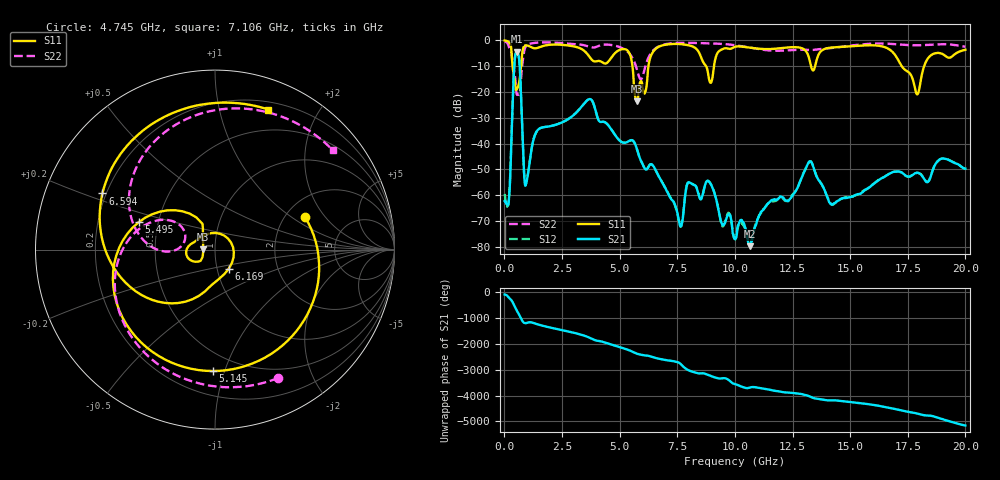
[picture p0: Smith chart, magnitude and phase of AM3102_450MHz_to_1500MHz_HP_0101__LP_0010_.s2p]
!Agilent Technologies,E8364B,MY43040894,A.07.50.67
!Agilent E8364B: A.07.50.67
!Date: Thursday, January 11, 2018 05:39:55
!Correction: S11(Full 2 Port(1,2))
!S21(Full 2 Port(1,2))
!S12(Full 2 Port(1,2))
!S22(Full 2 Port(1,2))
!S2P File: Measurements: S11, S21, S12, S22:
# Hz S  dB  R 50
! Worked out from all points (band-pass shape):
!   1601 points, 10 MHz to 20 GHz, reference 50 ohm
!   highest |S21| = -4.44 dB at 534.7 MHz (marker M1); lowest = -79.7 dB at 10.64 GHz (marker M2)
!   |S21| within 3 dB of the highest: 452.5 MHz to 642.6 MHz (190.1 MHz wide, 34.7 % of centre)
!   lowest |S11| = -23.6 dB at 5.745 GHz (marker M3), VSWR 1.14, Z = 43.8 + j0.156 ohm
!   |S11| at or under -10 dB: 355.8 MHz to 725.3 MHz (369.5 MHz wide, 68.3 % of centre); 5.555 GHz to 6.249 GHz (693.9 MHz wide, 11.8 % of centre); 17.24 GHz to 18.21 GHz (973.4 MHz wide, 5.49 % of centre)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
!   |S22| runs from -21.1 to -0.4 dB; largest |S21 - S12| = 0.0012
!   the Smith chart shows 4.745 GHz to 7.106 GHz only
!   S11 on the Smith chart (normalised r, x): 4.745 GHz: 2.54, +1.29; 5.145 GHz: 0.37, -0.91; 5.495 GHz: 0.39, +0.15; 6.169 GHz: 1.14, -0.25; 6.594 GHz: 0.19, +0.23; 7.106 GHz: 0.27, +1.42
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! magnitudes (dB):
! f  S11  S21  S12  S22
! 10 MHz  -0.1  -62.2  -59.5  -0.4
! 184.9 MHz  -0.6  -62.8  -63.2  -2.3
! 534.7 MHz  -18.6  -4.4  -4.4  -20.8
! 947 MHz  -1.9  -55.5  -55.2  -2.2
! 1.434 GHz  -3.0  -34.9  -34.9  -0.9
! 3.346 GHz  -3.4  -25.8  -25.7  -1.7
! 4.745 GHz  -5.5  -36.0  -35.9  -2.0
! 5.145 GHz  -3.4  -39.6  -39.6  -3.2
! 5.495 GHz  -6.9  -38.7  -38.7  -6.0
! 5.745 GHz  -23.6  -42.0  -41.9  -11.2
! 6.169 GHz  -17.6  -50.1  -49.9  -8.5
! 6.594 GHz  -3.1  -50.9  -50.9  -2.9
! 6.682 GHz  -2.6  -52.4  -52.4  -2.4
! 7.106 GHz  -1.6  -59.4  -59.2  -1.3
! 8.868 GHz  -14.5  -54.7  -54.6  -1.2
! 10.01 GHz  -2.5  -77.0  -76.6  -1.9
! 10.64 GHz  -2.8  -79.7  -78.2  -2.8
! 13.34 GHz  -11.1  -47.5  -47.5  -3.8
! 14.24 GHz  -2.8  -63.6  -63.8  -2.9
! 16.68 GHz  -3.4  -51.8  -51.8  -1.3
! 17.9 GHz  -20.9  -51.3  -51.3  -1.9
! 20 GHz  -3.7  -49.7  -49.7  -2.5
